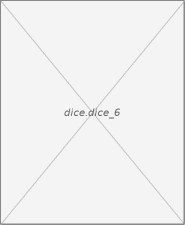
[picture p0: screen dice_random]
VISUALIZATION dice_random  // 185x225
VAR_IN_OUT
	invisible : ARRAY[1..6] OF BOOL;
END_VAR
    Image (0,0 185x225), invisible if: invisible[1], image: dice.dice_1
    Image (0,0 185x225), invisible if: invisible[2], image: dice.dice_2
    Image (0,0 185x225), invisible if: invisible[3], image: dice.dice_3
    Image (0,0 185x225), invisible if: invisible[4], image: dice.dice_4
    Image (0,0 185x225), invisible if: invisible[5], image: dice.dice_5
    Image (0,0 185x225), invisible if: invisible[6], image: dice.dice_6
END_VISUALIZATION
